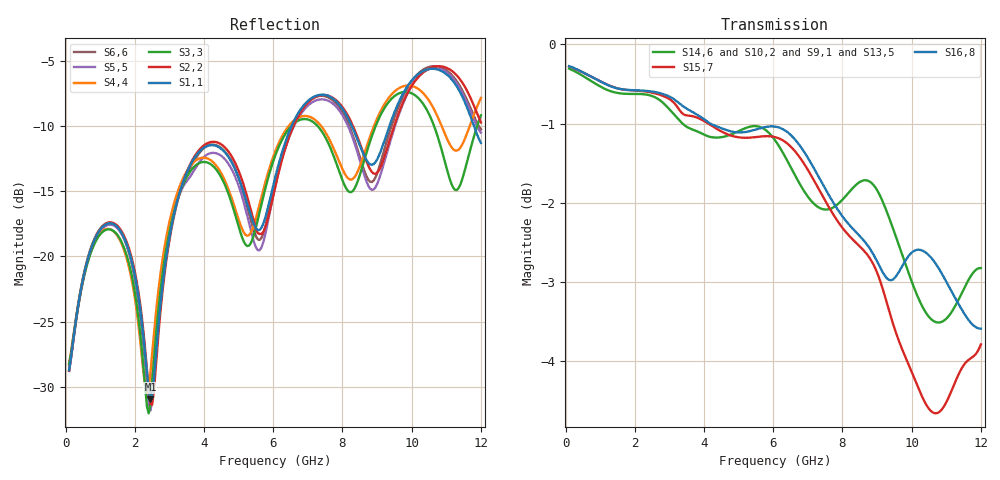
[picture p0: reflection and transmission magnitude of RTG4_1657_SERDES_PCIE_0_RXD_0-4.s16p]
! RTG4 1657 S-parameter file
! Microsemi Corporation (c) 2019
!Initial ver: Jul 30, 2019
! Port::PIN_NAME::NET_NAME::S-parameter ports::PORT SIDE
! Port1:--:SERDES_PCIE_0_RXD0_N_DIE::1::DIE
! Port2:--:SERDES_PCIE_0_RXD0_P_DIE::2::DIE
! Port3:AW4:SERDES_PCIE_0_RXD0_N_BGA::3::BGA
! Port4:AV4:SERDES_PCIE_0_RXD0_P_BGA::4::BGA
! Port5:--:SERDES_PCIE_0_RXD1_N_DIE::5::DIE
! Port6:--:SERDES_PCIE_0_RXD1_P_DIE::6::DIE
! Port7:BA5:SERDES_PCIE_0_RXD1_N_BGA::7::BGA
! Port8:AY5:SERDES_PCIE_0_RXD1_P_BGA::8::BGA
! Port9:--:SERDES_PCIE_0_RXD2_N_DIE::9::DIE
! Port10:--:SERDES_PCIE_0_RXD2_P_DIE::10::DIE
! Port11:BA7:SERDES_PCIE_0_RXD2_N_BGA::11::BGA
! Port12:AY7:SERDES_PCIE_0_RXD2_P_BGA::12::BGA
! Port13:--:SERDES_PCIE_0_RXD3_N_DIE::13::DIE
! Port14:--:SERDES_PCIE_0_RXD3_P_DIE::14::DIE
! Port15:BA9:SERDES_PCIE_0_RXD3_N_BGA::15::BGA
! Port16:AY9:SERDES_PCIE_0_RXD3_P_BGA::16::BGA
!TouchstoneFormatFlag = 1
! GNDNET
! NETSLIST
! User Comments:
! Touchstone file exported from HFSS 2018.2.0
!  File:  //LSI_Z840_SIM_PC/Simulation_Data/MASUMISU/Microsemi_190710/YBD197_150320_NETCHANGE_SERDES_PCIE_0_RXD.aedt
!  Generated:  9:31:11 ??  7 16, 2019
!  Design:  HFSSModel1
!  Project:  YBD197_150320_NETCHANGE_SERDES_PCIE_0_RXD
!  Setup:  Setup1
!  Solution:  Sweep
! Terminal data exported
! Port[1] = SERDES_PCIE_0_RXD0_N_DIE
! Port[2] = SERDES_PCIE_0_RXD0_P_DIE
! Port[3] = SERDES_PCIE_0_RXD1_N_DIE
! Port[4] = SERDES_PCIE_0_RXD1_P_DIE
! Port[5] = SERDES_PCIE_0_RXD2_N_DIE
! Port[6] = SERDES_PCIE_0_RXD2_P_DIE
! Port[7] = SERDES_PCIE_0_RXD3_N_DIE
! Port[8] = SERDES_PCIE_0_RXD3_P_DIE
! Port[9] = SERDES_PCIE_0_RXD0_N_BGA
! Port[10] = SERDES_PCIE_0_RXD0_P_BGA
! Port[11] = SERDES_PCIE_0_RXD1_N_BGA
! Port[12] = SERDES_PCIE_0_RXD1_P_BGA
! Port[13] = SERDES_PCIE_0_RXD2_N_BGA
! Port[14] = SERDES_PCIE_0_RXD2_P_BGA
! Port[15] = SERDES_PCIE_0_RXD3_N_BGA
! Port[16] = SERDES_PCIE_0_RXD3_P_BGA
# GHZ S DB R 50.000000
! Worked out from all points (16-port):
!   239 points, 100 MHz to 12 GHz, reference 50 ohm
!   strongest paths, dB at 100 MHz, 3.05 GHz, 6.05 GHz, 9.05 GHz, 12 GHz:
!     S16,8: -0.3, -0.7, -1.0, -2.8, -3.6
!     S15,7: -0.3, -0.7, -1.2, -2.9, -3.8
!     S14,6: -0.3, -0.8, -1.2, -1.9, -2.8
!     S10,2: -0.3, -0.7, -1.2, -2.0, -3.0
!     S9,1: -0.3, -0.7, -1.3, -2.0, -3.1
!     S13,5: -0.3, -0.8, -1.3, -2.2, -3.1
!   lowest |S11| = -31.0 dB at 2.45 GHz (marker M1), VSWR 1.06, Z = 51.9 + j2.16 ohm
!   |S11| at or under -10 dB: start of sweep to 6.526 GHz; 8.273 GHz to 9.354 GHz (1.081 GHz wide, 12.3 % of centre); 11.8 GHz to end of sweep
